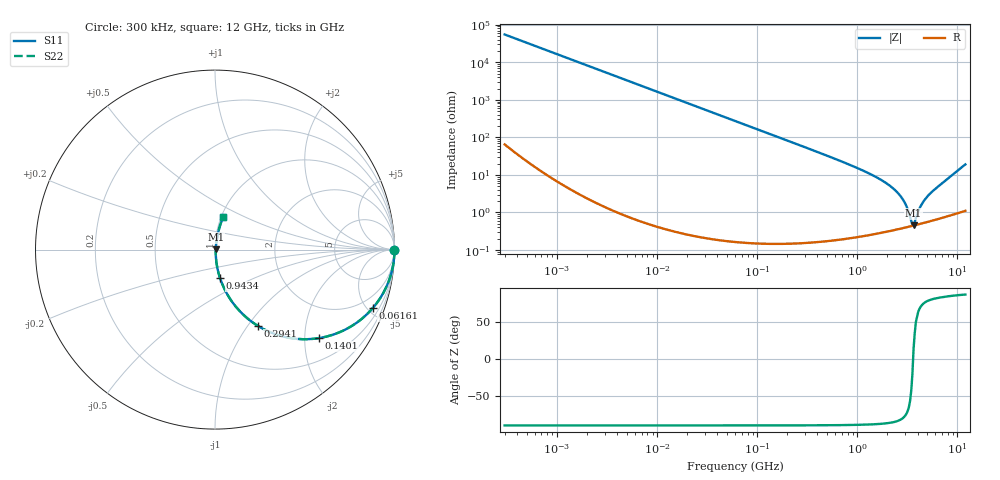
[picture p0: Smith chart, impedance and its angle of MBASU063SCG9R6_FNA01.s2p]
! MBASU063SCG9R6_FNA01  S-PARAMETER MODEL  ( General Type )
! Model Generated by TAIYO YUDEN Corporation (http://www.ty-top.com)
! Version 1.0
! TAIYO YUDEN Control No. 130801
! Copyright(c) 2013 TAIYO YUDEN CO.,LTD. All Rights Reserved.
! Product Description (link to TY-COMPAS)
! https://ds.yuden.co.jp/TYCOMPAS/or/detail?pn=MBASU063SCG9R6DFNA01&u=M
! Products Name : Multilayer Ceramic Capacitors
! Characteristics :
!  Capacitance : 9.6 pF , Rated Voltage : 50V , TCC : CG / C0G
!  Case Size : 0.6 x 0.3 / 0.024 x 0.012 [mm/inch] , Thickness : 0.3 / 0.012 [mm/inch]
!  (Conditions: Temperature = 25 degC , DC Bias Current/Voltage = 0A / 0V)
! External Node Assignments :
!  1  o---| |---o  2
! GND o---------o GND
! Frequency Range : 0.3MHz  -  12000MHz  [ 401 STEP ]
# MHz S RI R 50
! Freq[MHz].  S11 Real  S11 Imag  S21 Real  S21 Imag  S12 Real  S12 Imag  S22 Real  S22 Imag
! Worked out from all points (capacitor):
!   401 points, 300 kHz to 12 GHz, reference 50 ohm
!   read as one part in series: C = 9.64 pF near 316.3 kHz
!   lowest |Z| = 460 mohm at 3.643 GHz (marker M1)
!   series resonance near 3.606 GHz, so ESL is about 200 pH
!   S11 on the Smith chart (normalised r, x): 300 kHz: open; 61.61 MHz: 1.00, -5.36; 140.1 MHz: 1.00, -2.36; 294.1 MHz: 1.00, -1.12; 943.4 MHz: 1.00, -0.33; 12 GHz: 1.02, +0.38
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0.3  1 -0.00182  5.44e-06 0.00182  5.44e-06 0.00182  1 -0.00182
1.769972  0.9999 -0.0107  0.000118 0.0107  0.000118 0.0107  0.9999 -0.0107
10.44266  0.996 -0.063  0.004 0.063  0.004 0.063  0.996 -0.063
26.39317  0.975 -0.1558  0.025 0.1558  0.025 0.1558  0.975 -0.1558
60  0.8832 -0.3208  0.1168 0.3208  0.1168 0.3208  0.8832 -0.3208
61.61074  0.8777 -0.3274  0.1223 0.3274  0.1223 0.3274  0.8777 -0.3274
91.67136  0.7641 -0.4241  0.2359 0.4241  0.2359 0.4241  0.7641 -0.4241
140.0606  0.5809 -0.4928  0.4191 0.4928  0.4191 0.4928  0.5809 -0.4928
197.6437  0.4099 -0.4909  0.5901 0.4909  0.5901 0.4909  0.4099 -0.4909
294.0765  0.238 -0.4245  0.762 0.4245  0.762 0.4245  0.238 -0.4245
353.9943  0.1768 -0.3798  0.8232 0.3798  0.8232 0.3798  0.1768 -0.3798
943.3804  0.0279 -0.1582  0.9721 0.1582  0.9721 0.1582  0.0279 -0.1582
1519.776  0.0105 -0.0883  0.9895 0.0883  0.9895 0.0883  0.0105 -0.0883
2088.533  0.0059 -0.0522  0.9941 0.0522  0.9941 0.0522  0.0059 -0.0522
2795.104  0.00432 -0.0235  0.9957 0.0235  0.9957 0.0235  0.00432 -0.0235
3107.553  0.00421 -0.0137  0.9958 0.0137  0.9958 0.0137  0.00421 -0.0137
3454.93  0.00432 -0.00401  0.9957 0.00401  0.9957 0.00401  0.00432 -0.00401
3642.919  0.00446 0.00103  0.9955 -0.00103  0.9955 -0.00103  0.00446 0.00103
3740.715  0.00455 0.00306  0.9955 -0.00306  0.9955 -0.00306  0.00455 0.00306
4385.161  0.00529 0.0154  0.9947 -0.0154  0.9947 -0.0154  0.00529 0.0154
5140.631  0.00645 0.0281  0.9936 -0.0281  0.9936 -0.0281  0.00645 0.0281
12000  0.0448 0.1798  0.9552 -0.1798  0.9552 -0.1798  0.0448 0.1798
